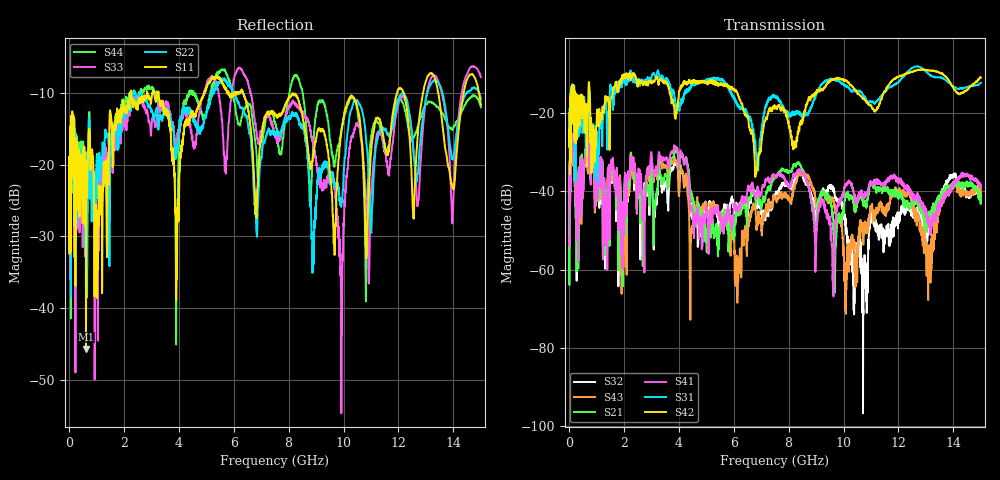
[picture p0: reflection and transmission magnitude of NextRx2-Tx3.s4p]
! FILE: N:\QM 2007\Prüfprotokolle\Highspeed\Konfektionierte Ltg\L45593-D106\D30\8216\0002\Next\NextRx2-Tx3.s4p
# MHz S DB R 50.00
! FREQ  S11  S12  S13  S14
!  S21  S22  S23  S24
!  S31  S32  S33  S34
!  S41  S42  S43  S44
!  DB  ANG  DB  ANG  DB  ANG  DB  ANG
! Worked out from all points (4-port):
!   2999 points, 10 MHz to 15 GHz, reference 50 ohm
!   strongest paths, dB at 10 MHz, 3.755 GHz, 7.505 GHz, 11.26 GHz, 15 GHz:
!     S42: -24.3, -16.7, -18.5, -18.7, -10.9
!     S31: -24.1, -14.4, -15.6, -16.5, -12.3
!     S41: -51.9, -30.1, -36.0, -38.1, -38.7
!     S21: -43.3, -31.6, -36.3, -38.8, -42.1
!     S43: -43.6, -32.7, -41.3, -45.1, -40.6
!     S32: -52.4, -34.0, -40.7, -49.3, -41.5
!   lowest |S11| = -45.7 dB at 625 MHz (marker M1), VSWR 1.01, Z = 49.5 - j0.0236 ohm
!   |S11| at or under -10 dB: start of sweep to 2.229 GHz; 3.27 GHz to 4.927 GHz (1.657 GHz wide, 40.4 % of centre); 6.338 GHz to 11.95 GHz (5.609 GHz wide, 61.4 % of centre)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
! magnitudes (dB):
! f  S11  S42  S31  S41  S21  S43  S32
! 10 MHz  -18.9  -24.3  -24.1  -51.9  -43.3  -43.6  -52.4
! 625 MHz  -45.7  -18.7  -24.0  -32.7  -33.6  -32.9  -33.7
! 6.11 GHz  -10.0  -14.6  -17.6  -44.2  -45.8  -59.7  -44.3
! 6.83 GHz  -27.5  -34.9  -30.3  -40.5  -41.9  -49.8  -42.4
! 9.91 GHz  -15.7  -11.2  -12.3  -42.0  -47.7  -47.7  -42.7
! 10.74 GHz  -21.6  -16.4  -15.6  -40.8  -43.0  -51.1  -63.0
! 15 GHz  -11.7  -10.9  -12.3  -38.7  -42.1  -40.6  -41.5
